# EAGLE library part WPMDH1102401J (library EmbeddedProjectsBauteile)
MagI³C-VDRM Variable Step Down Regulator
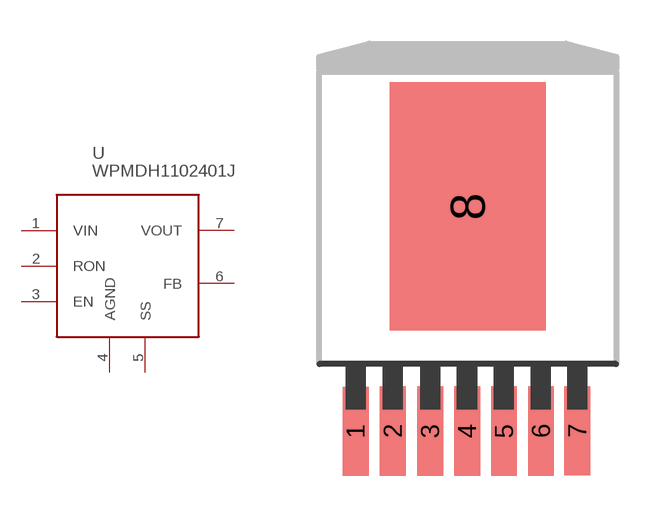
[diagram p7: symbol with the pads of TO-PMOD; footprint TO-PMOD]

Designator prefix -

## WPMDH1102401J  [TO-PMOD]
1  VIN  in
2  RON  in
3  EN  in
4  AGND  pas
5  SS
6  FB
7  VOUT  out

## Footprint TO-PMOD (pad centres in mm)
smd 0.89 x 3.06: 1 -3.834,-7.381; 2 -2.554,-7.371; 3 -1.274,-7.371; 4 -0.004,-7.371; 5 1.266,-7.371; 6 2.536,-7.371; 7 3.786,-7.361
smd 5.35 x 8.54: 8 0.02,0.36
